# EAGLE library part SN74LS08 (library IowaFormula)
Quad 2-input AND gate SN74LS08 Google Drive Datasheet
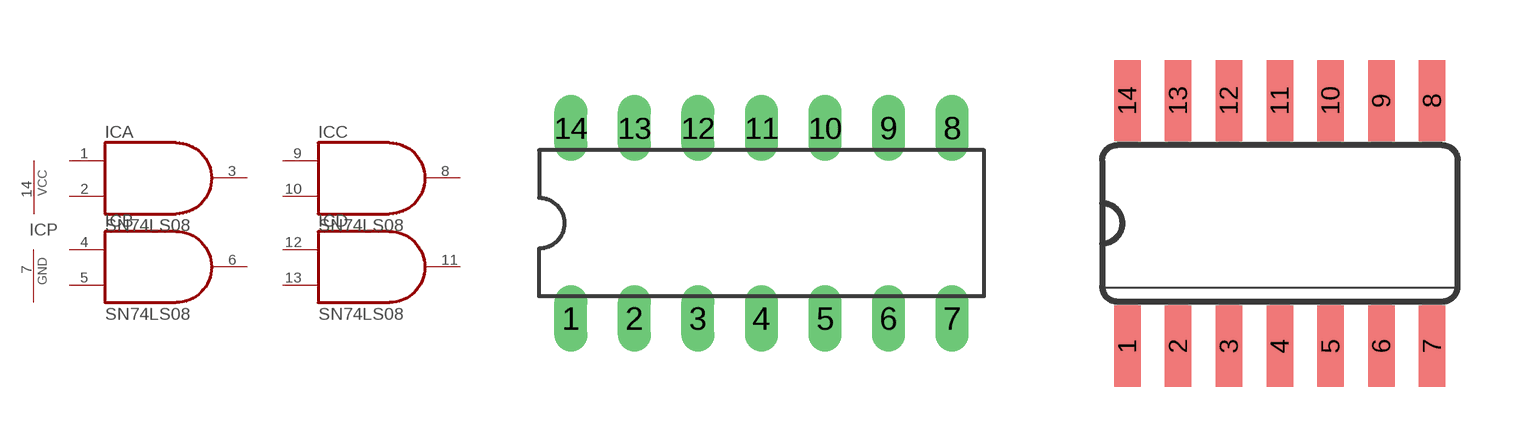
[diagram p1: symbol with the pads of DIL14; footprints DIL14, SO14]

Designator prefix IC; gates A=7408 B=7408 C=7408 D=7408 P=PWRN-2

## SN74LS08ALSN, SN74LS08ASN, SN74LS08LSN, SN74LS08SN  [DIL14]
1  A:I0  in
2  A:I1  in
3  A:O  out
4  B:I0  in
5  B:I1  in
6  B:O  out
7  P:GND  pwr
8  C:O  out
9  C:I0  in
10  C:I1  in
11  D:O  out
12  D:I0  in
13  D:I1  in
14  P:VCC  pwr

## SN74LS08ALSD, SN74LS08ASD, SN74LS08LSD, SN74LS08SD  [SO14]
Pads as for DIL14

## Footprint DIL14 (pad centres in mm)
Dual In Line Package
drill 0.813 long: 1 -7.62,-3.81; 2 -5.08,-3.81; 3 -2.54,-3.81; 4 0,-3.81; 5 2.54,-3.81; 6 5.08,-3.81; 7 7.62,-3.81; 8 7.62,3.81; 9 5.08,3.81; 10 2.54,3.81; 11 0,3.81; 12 -2.54,3.81; 13 -5.08,3.81; 14 -7.62,3.81

## Footprint SO14 (pad centres in mm)
Small Outline package 150 mil
smd 0.66 x 2.032: 1 -3.81,-3.073; 2 -2.54,-3.073; 3 -1.27,-3.073; 4 0,-3.073; 5 1.27,-3.073; 6 2.54,-3.073; 7 3.81,-3.073; 8 3.81,3.073; 9 2.54,3.073; 10 1.27,3.073; 11 0,3.073; 12 -1.27,3.073; 13 -2.54,3.073; 14 -3.81,3.073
